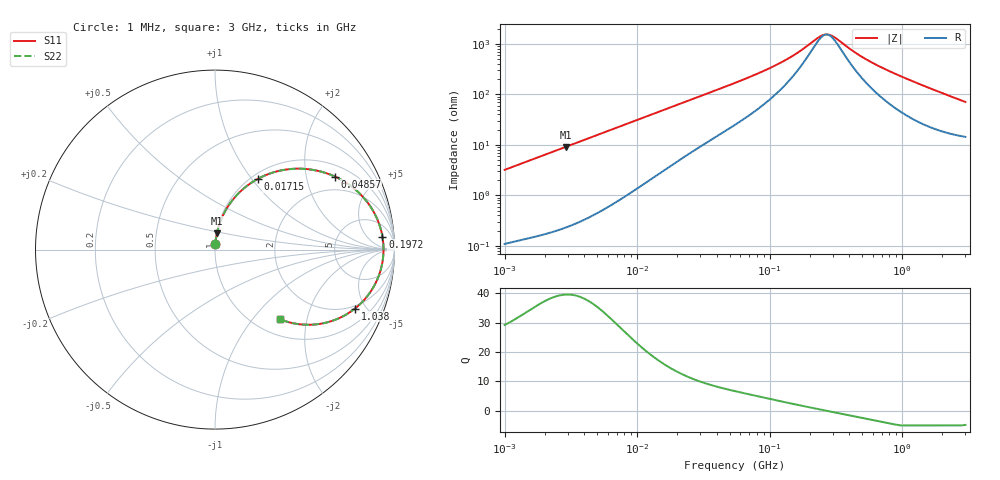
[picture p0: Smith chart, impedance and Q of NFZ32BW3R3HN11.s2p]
! NFZ32BW3R3HN11
# Hz S RI R 50
!Freq.(Hz) S11(Real) S11(Imag) S21(Real) S21(Imag) S12(Real) S12(Imag) S22(Real) S22(Imag)
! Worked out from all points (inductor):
!   401 points, 1 MHz to 3 GHz, reference 50 ohm
!   read as one part in series: L = 507 nH near 1.041 MHz
!   highest Q = 39.6 at 2.889 MHz (marker M1), where L = 503 nH
!   self-resonance near 269.2 MHz
!   S11 on the Smith chart (normalised r, x): 1 MHz: 1.00, +0.06; 17.15 MHz: 1.07, +1.07; 48.57 MHz: 1.41, +2.96; 197.2 MHz: 13, +15; 1.038 GHz: 1.81, -4.19; 3 GHz: 1.29, -1.39
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1000000  0.00211 0.0319  0.9979 -0.0319  0.9979 -0.0319  0.00211 0.0319
2888807  0.0105 0.0901  0.9895 -0.0901  0.9895 -0.0901  0.0105 0.0901
3823119  0.0173 0.1181  0.9827 -0.1181  0.9827 -0.1181  0.0173 0.1181
8179831  0.0698 0.2368  0.9302 -0.2368  0.9302 -0.2368  0.0698 0.2368
1.461624e7  0.1867 0.3614  0.8133 -0.3614  0.8133 -0.3614  0.1867 0.3614
1.71545e7  0.2371 0.3933  0.7629 -0.3933  0.7629 -0.3933  0.2371 0.3933
2.886629e7  0.4477 0.4507  0.5523 -0.4507  0.5523 -0.4507  0.4477 0.4507
4.857399e7  0.669 0.4067  0.331 -0.4067  0.331 -0.4067  0.669 0.4067
5.477226e7  0.7127 0.384  0.2873 -0.384  0.2873 -0.384  0.7127 0.384
7.852918e7  0.8183 0.3  0.1817 -0.3  0.1817 -0.3  0.8183 0.3
1.148668e8  0.8885 0.2021  0.1115 -0.2021  0.1115 -0.2021  0.8885 0.2021
1.520175e8  0.9181 0.1323  0.0819 -0.1323  0.0819 -0.1323  0.9181 0.1323
1.971969e8  0.9331 0.0708  0.0669 -0.0708  0.0669 -0.0708  0.9331 0.0708
2.094008e8  0.9352 0.057  0.0648 -0.057  0.0648 -0.057  0.9352 0.057
2.507343e8  0.9386 0.016  0.0614 -0.016  0.0614 -0.016  0.9386 0.016
2.716345e8  0.9389 -0.00205  0.0611 0.00205  0.0611 0.00205  0.9389 -0.00205
2.884452e8  0.9386 -0.0156  0.0614 0.0156  0.0614 0.0156  0.9386 -0.0156
4.951867e8  0.9139 -0.142  0.0861 0.142  0.0861 0.142  0.9139 -0.142
8.005644e8  0.8446 -0.2645  0.1554 0.2645  0.1554 0.2645  0.8446 -0.2645
1.038491e9  0.779 -0.3291  0.221 0.3291  0.221 0.3291  0.779 -0.3291
1.782824e9  0.5764 -0.415  0.4236 0.415  0.4236 0.415  0.5764 -0.415
3e9  0.3609 -0.3875  0.6391 0.3875  0.6391 0.3875  0.3609 -0.3875
